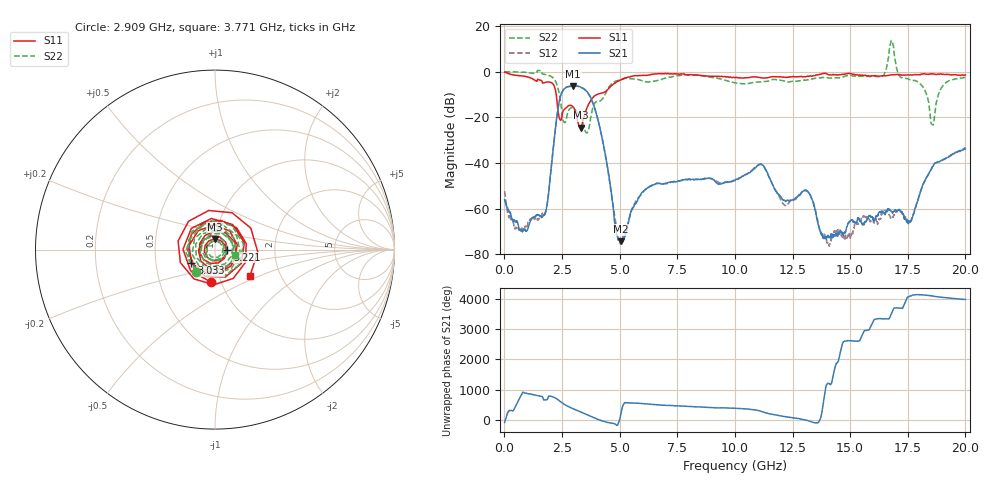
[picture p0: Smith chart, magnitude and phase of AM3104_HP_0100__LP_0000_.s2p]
!Created with skrf (http://scikit-rf.org).
# Hz S RI R 50.0
!freq ReS11 ImS11 ReS21 ImS21 ReS12 ImS12 ReS22 ImS22
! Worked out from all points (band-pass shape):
!   1601 points, 10 MHz to 20 GHz, reference 50 ohm
!   highest |S21| = -6.21 dB at 2.984 GHz (marker M1); lowest = -74.4 dB at 5.045 GHz (marker M2)
!   |S21| within 3 dB of the highest: 2.489 GHz to 3.617 GHz (1.128 GHz wide, 37 % of centre)
!   lowest |S11| = -24.6 dB at 3.321 GHz (marker M3), VSWR 1.13, Z = 49.6 + j5.89 ohm
!   |S11| at or under -10 dB: 2.249 GHz to 4.023 GHz (1.773 GHz wide, 56.6 % of centre)
!   |S22| runs from -26.9 to 13.7 dB; largest |S21 - S12| = 0.027
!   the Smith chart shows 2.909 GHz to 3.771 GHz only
!   S11 on the Smith chart (normalised r, x): 2.909 GHz: 0.90, -0.33; 3.033 GHz: 0.76, -0.12; 3.221 GHz: 1.15, -0.00; 3.771 GHz: 1.40, -0.44
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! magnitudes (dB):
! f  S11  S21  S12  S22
! 10 MHz  -0.3  -56.1  -52.4  0.0
! 522.2 MHz  -1.6  -65.5  -69.2  -0.1
! 1.709 GHz  -4.9  -63.0  -62.2  -1.1
! 2.396 GHz  -20.6  -12.3  -12.4  -10.6
! 2.909 GHz  -14.8  -6.3  -6.4  -15.7
! 2.984 GHz  -15.5  -6.2  -6.2  -15.9
! 3.033 GHz  -16.4  -6.3  -6.3  -16.2
! 3.221 GHz  -23.2  -6.4  -6.5  -18.8
! 3.321 GHz  -24.6  -6.8  -6.9  -20.0
! 3.346 GHz  -24.3  -6.9  -7.0  -20.6
! 3.771 GHz  -12.3  -12.0  -12.0  -18.9
! 5.045 GHz  -3.6  -74.4  -75.4  -3.6
! 6.682 GHz  -0.9  -48.9  -48.9  -3.8
! 10.01 GHz  -2.6  -47.6  -47.7  -4.9
! 11.14 GHz  -2.7  -40.6  -40.7  -4.5
! 12.13 GHz  -2.4  -56.4  -58.2  -4.0
! 13.34 GHz  -2.0  -55.9  -55.7  -3.2
! 14.08 GHz  -1.4  -72.7  -75.2  -2.8
! 16.68 GHz  -1.5  -60.7  -62.6  7.2
! 17.6 GHz  -1.4  -66.0  -65.1  -3.5
! 18.56 GHz  -0.9  -41.7  -41.8  -23.2
! 20 GHz  -1.4  -33.9  -33.3  -2.5
